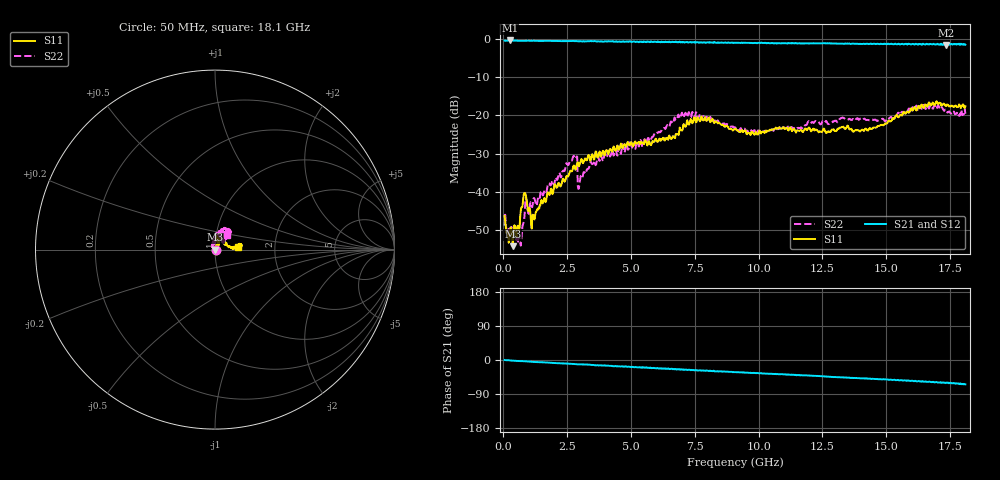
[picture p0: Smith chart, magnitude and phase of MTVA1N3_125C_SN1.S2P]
! Network Analyzer HP8720D.06.14 Serial No. US36140669
! 10 Jan 2005  15:26:23
! Frequency  S11  S21  S12  S22
# HZ  S  DB R 50
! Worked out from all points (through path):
!   801 points, 50 MHz to 18.1 GHz, reference 50 ohm
!   highest |S21| = -0.46 dB at 253.1 MHz (marker M1); lowest = -1.6 dB at 17.33 GHz (marker M2)
!   group delay of S21, straight-line fit = 9.41 ps
!   lowest |S11| = -54.1 dB at 365.9 MHz (marker M3), VSWR 1.00, Z = 50.2 - j0.0165 ohm
!   |S11| at or under -10 dB: start of sweep to end of sweep
!   |S22| runs from -54.0 to -17.2 dB; largest |S21 - S12| = 0.024
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5e7  -46.25 -32.2  -0.50 0.0  -0.50 -0.5  -48.79 3.7
2.530625e8  -51.21 -0.4  -0.46 -1.0  -0.46 -1.4  -50.25 -25.3
3.65875e8  -54.13 -4.8  -0.47 -1.8  -0.46 -1.9  -51.54 -28.0
6.36625e8  -49.28 59.6  -0.54 -3.0  -0.52 -3.1  -52.85 -17.3
8.17125e8  -40.34 39.4  -0.54 -3.4  -0.53 -3.5  -47.16 -73.7
1.178125e9  -46.20 41.1  -0.52 -5.1  -0.53 -5.2  -41.76 145.1
2.689812e9  -34.56 58.3  -0.60 -10.3  -0.59 -10.6  -31.70 122.3
2.802625e9  -33.79 50.5  -0.66 -10.8  -0.62 -11.2  -31.24 117.5
3.005688e9  -32.48 73.1  -0.65 -11.6  -0.67 -11.8  -36.92 135.5
3.073375e9  -31.50 66.4  -0.67 -11.5  -0.61 -12.0  -36.13 129.3
3.772812e9  -29.44 59.1  -0.73 -14.2  -0.65 -14.3  -31.89 119.7
6.074188e9  -26.79 68.9  -0.80 -22.6  -0.80 -22.4  -24.46 94.0
7.202312e9  -21.27 79.5  -0.85 -26.1  -0.87 -25.9  -20.48 67.1
7.969438e9  -21.43 75.5  -0.97 -27.9  -0.92 -28.6  -20.39 51.0
9.075e9  -23.58 83.6  -1.07 -31.9  -1.02 -32.2  -23.19 43.3
9.954938e9  -25.02 82.1  -1.11 -34.2  -1.09 -35.0  -24.14 44.4
1.209838e10  -23.88 61.3  -1.19 -41.5  -1.18 -41.8  -21.73 66.1
1.403875e10  -23.75 29.5  -1.38 -48.5  -1.34 -48.7  -20.94 69.3
1.509919e10  -21.33 10.9  -1.38 -52.3  -1.27 -52.1  -20.96 75.6
1.640781e10  -17.31 7.2  -1.52 -55.9  -1.37 -56.3  -18.14 61.1
1.733288e10  -17.40 7.7  -1.63 -59.6  -1.64 -60.6  -18.51 45.3
1.81e10  -17.64 7.3  -1.56 -64.4  -1.54 -65.4  -19.56 52.0
